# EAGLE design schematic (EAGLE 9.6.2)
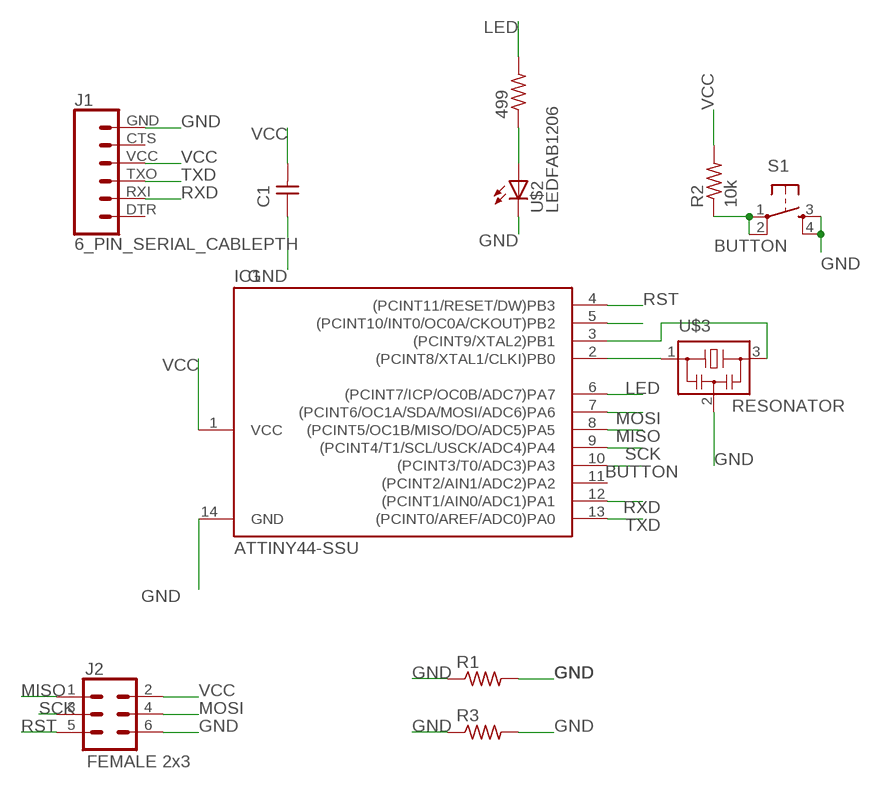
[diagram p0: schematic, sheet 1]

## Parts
499  RES-US1206FAB  [R1206FAB]
C1  CAP-UNPOLARIZEDFAB  [C1206FAB]
IC1  ATTINY44-SSU  [SOIC14]
J1  6_PIN_SERIAL_CABLEPTH  [FTDI_BASIC]
J2  FEMALE 2x3  CONN_03X2FEMALE  [2X3]
R1  RES-US1206FAB  [R1206FAB]
R2  10k  RES-US1206FAB  [R1206FAB]
R3  RES-US1206FAB  [R1206FAB]
S1  6MM_SWITCH6MM_SWITCH  [6MM_SWITCH]
U$2  LEDFAB1206  [LED1206FAB]
U$3  RESONATOR  [EFOBM]

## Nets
BUTTON: IC1.10((PCINT3/T0/ADC3)PA3) R2.1 S1.1(P) S1.2(P1)
GND: C1.1 IC1.14(GND) J1.GND J2.6 R1.1 R1.2 R3.1 R3.2 S1.3(S) S1.4(S1) U$2.2(C) U$3.2
LED: 499.2 IC1.6((PCINT7/ICP/OC0B/ADC7)PA7)
MISO: IC1.8((PCINT5/OC1B/MISO/DO/ADC5)PA5) J2.1
MOSI: IC1.7((PCINT6/OC1A/SDA/MOSI/ADC6)PA6) J2.4
N$1: IC1.5((PCINT10/INT0/OC0A/CKOUT)PB2)
N$4: IC1.2((PCINT8/XTAL1/CLKI)PB0) U$3.1
N$5: IC1.3((PCINT9/XTAL2)PB1) U$3.3
N$6: 499.1 U$2.1(A)
RST: IC1.4((PCINT11/RESET/DW)PB3) J2.5
RXD: IC1.12((PCINT1/AIN0/ADC1)PA1) J1.RXI
SCK: IC1.9((PCINT4/T1/SCL/USCK/ADC4)PA4) J2.3
TXD: IC1.13((PCINT0/AREF/ADC0)PA0) J1.TXO
VCC: C1.2 IC1.1(VCC) J1.VCC J2.2 R2.2
Unconnected: IC1.11((PCINT2/AIN1/ADC2)PA2) J1.CTS J1.DTR

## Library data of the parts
499 R1-R3 = fab:RES-US: Resistor (US Symbol)
C1 = fab:CAP-UNPOLARIZED
IC1 = fab:ATTINY44
J1 = SparkFun-Connectors:6_PIN_SERIAL_CABLE: 6-pin header connection for use with the "FTDI BASIC" pinout - CABLE SIDE. Also known as "Arduino Serial Program Header". This is used on a design to provide a 6-pin connection point for serial communication usually from a USB cable (D+/D-) to these headers (RX/TX). It also has the remaining pins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
J2 = SparkFun-Connectors:CONN_03X2: Multi connection point. Often used as Generic Header-pin footprint for 0.1 inch spaced/style header connections You can populate with any combo of single row headers, but if you'd like an exact match, check these: Header - 2x3 (Male, 0.1") (PRT-12807) Header - 2x3 (Female, 0.1") (PRT-13010) 2x3 Pin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; PROD_ID: CONN-11566
S1 = fab:6MM_SWITCH: OMRON SWITCH
U$2 = fab:LED: LED
U$3 = fab:RESONATOR

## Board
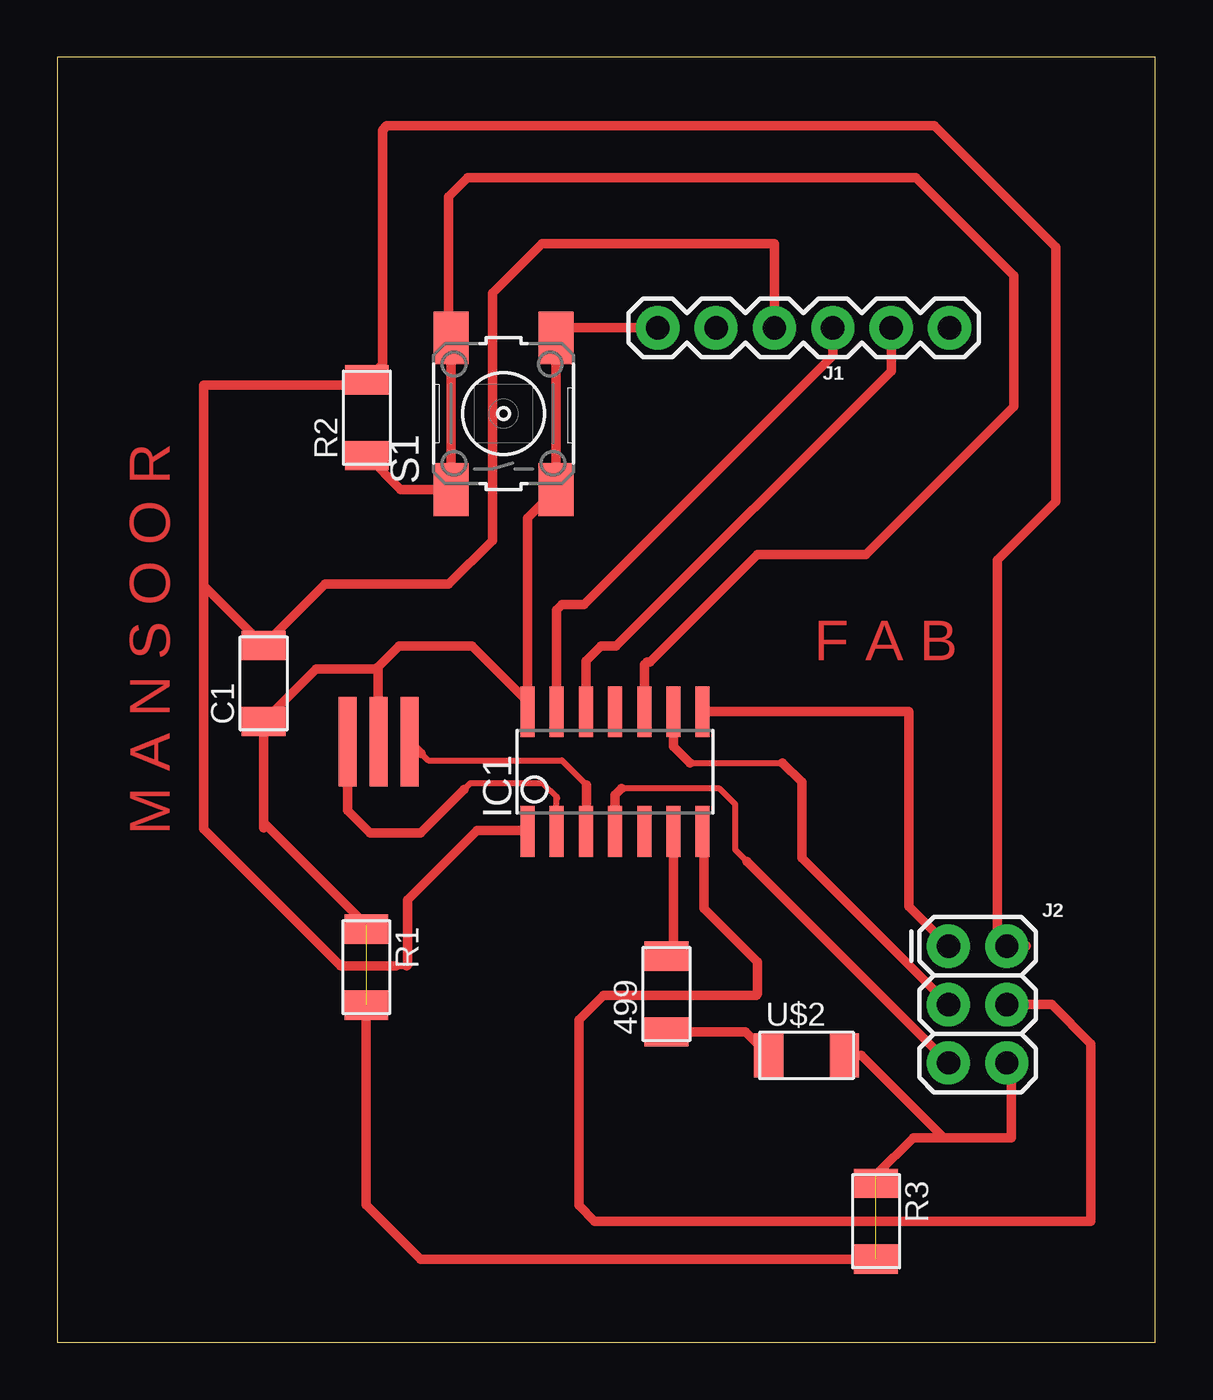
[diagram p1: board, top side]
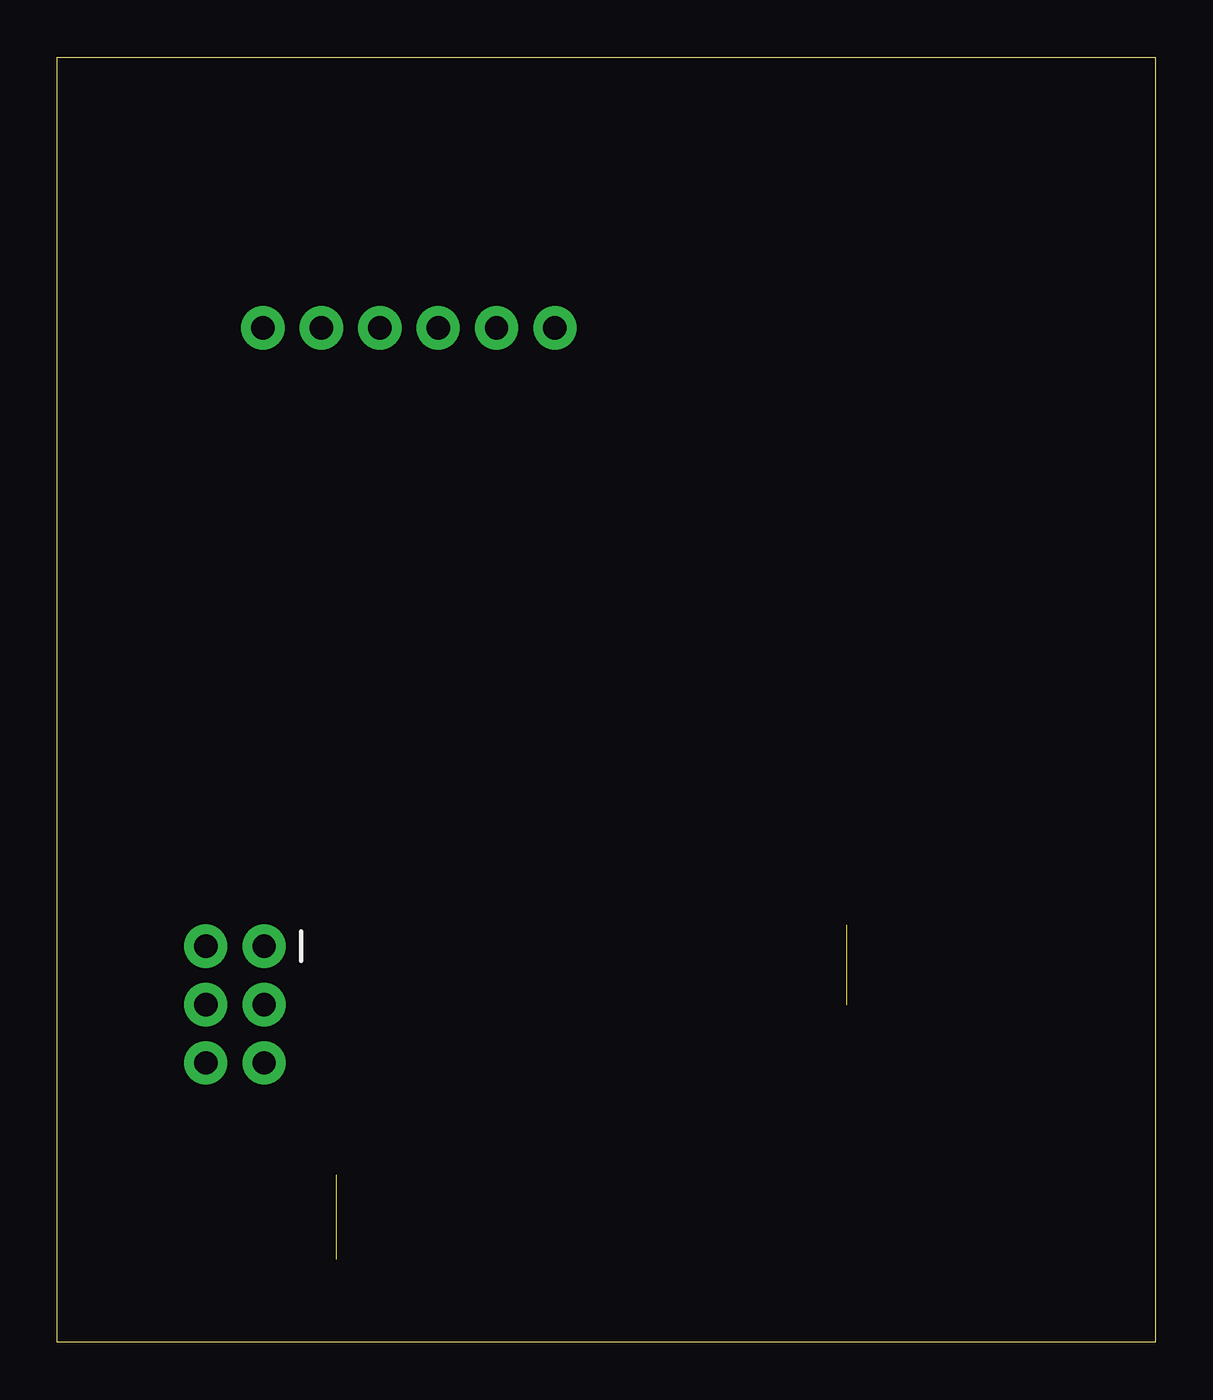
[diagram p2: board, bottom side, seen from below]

Size 47.75 x 55.88 mm. Coordinates in mm from the lower left corner, seen from the top.
Outline: 0,0 47.75,0 47.75,55.88 0,55.88 0,0
Copper layers (1*16): Top 0.035mm / dielectric 1.5mm / Bottom 0.035mm
Design rules "default *": minimum track width 6mil, minimum drill 0.35mm, track to track 16mil, track to pad 8mil, pad to pad 8mil, via to via 8mil, smd to smd 8mil, copper to edge 40mil, drill to drill 6mil, minimum pad ring 10mil, minimum via ring 8mil, stop-mask expansion 4mil, vias tented up to drill 0mil, thermal gap 10mil

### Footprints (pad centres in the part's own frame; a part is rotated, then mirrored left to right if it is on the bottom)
R1206FAB = smd 1.27 x 1.905: 1 -1.651,0; 2 1.651,0
C1206FAB = smd 1.27 x 1.905: 1 -1.651,0; 2 1.651,0
SOIC14 = smd 0.61 x 2.21: 1 -3.81,-2.603; 2 -2.54,-2.603; 3 -1.27,-2.603; 4 0,-2.603; 5 1.27,-2.603; 6 2.54,-2.603; 7 3.81,-2.603; 8 3.81,2.603; 9 2.54,2.603; 10 1.27,2.603; 11 0,2.603; 12 -1.27,2.603; 13 -2.54,2.603; 14 -3.81,2.603
FTDI_BASIC = drill 1.016 pad 1.88: CTS 10.16,0; DTR 0,0; GND 12.7,0; RXI 2.54,0; TXO 5.08,0; VCC 7.62,0
2X3 = drill 1.016 pad 1.88: 1 0,0; 2 0,2.54; 3 2.54,0; 4 2.54,2.54; 5 5.08,0; 6 5.08,2.54
6MM_SWITCH = smd 2.286 x 1.524: 1 -3.302,2.286; 2 3.302,2.286; 3 -3.302,-2.286; 4 3.302,-2.286
LED1206FAB = smd 1.27 x 1.905: 1 -1.651,0; 2 1.651,0
EFOBM = smd 0.8 x 3.9: 1 -1.35,0; 2 0,0; 3 1.35,0

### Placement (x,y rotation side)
499  26.49,15.14 90 top
C1  8.97,28.65 90 top
IC1  24.26,24.82 0 top
J1  38.81,44.12 180 top
J2  38.76,17.22 270 top
R1  13.44,16.31 270 top
R2  13.46,40.21 90 top
R3  35.61,5.26 270 top
S1  19.41,40.39 90 top
U$2  32.59,12.47 0 top
U$3  13.97,26.11 0 top

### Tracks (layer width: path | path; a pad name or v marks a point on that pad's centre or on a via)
BUTTON
  Top 0.406: 25.53,28.47 IC1.10 25.53,29.46 25.65,29.59 25.78,29.59 30.45,34.27 35.18,34.27 41.6,40.69 41.6,46.38 37.34,50.65 17.83,50.65 17,49.82 17,43.8 S1.2 | S1.2 17.12,43.92 | S1.2 S1.1 14.94,37.08 R2.1
GND  (4 unrouted)
  Top 0.406: U$3.2 13.96,26.13 13.96,29.37 | 41.81,11.63 41.5,11.94 | J1.GND 22.12,44.12 S1.4 S1.3 20.45,35.84 IC1.14 20.45,27.86 18.03,30.28 14.86,30.28 13.96,29.37 | 13.96,29.37 13.87,29.29 11.25,29.29 C1.1 8.97,22.61 | U$2.2 34.98,12.47 38.56,8.89 | 38.56,8.89 41.5,8.89 41.5,11.94 | 41.5,11.94 J2.6 | 38.56,8.89 37.24,8.89 35.61,7.26 | 8.97,22.35 8.97,22.61 | 8.97,22.61 13.44,18.14 | R1.2 13.44,5.97 15.8,3.61 R3.2
LED
  Top 0.406: 499.2 26.8,17.09 IC1.6
MISO
  Top 0.406: J2.1 37.03,18.95 37.03,27.42 IC1.8
MOSI
  Top 0.406: J2.4 43.26,14.68 44.96,12.98 44.96,5.26 23.37,5.26 22.68,5.94 22.68,14.02 23.75,15.09 30.4,15.09 30.45,15.14 30.45,16.54 28.12,18.87 28.12,22.16 IC1.7
N$4
  Top 0.254: IC1.2 21.72,23.62 | 21.72,23.62 21.74,23.65 | 21.72,23.62 21.72,23.72 21.13,24.31 17.96,24.31 17.68,24.03
  Top 0.406: U$3.1 12.63,23.13 13.61,22.15 15.8,22.15 17.68,24.03
N$5
  Top 0.254: 15.83,25.6 16.13,25.3 21.95,25.3 23.01,24.23
  Top 0.406: U$3.3 15.83,25.6 | 23.01,24.23 23.01,22.24 IC1.3
N$6
  Top 0.406: U$2.1 29.92,13.49 499.1
RST  (via drill 0.35)
  Top 0.254: 30,20.9 29.49,21.41 29.49,23.39 28.8,24.08 24.54,24.08
  Top 0.406: J2.5 30,20.9 | 24.54,24.08 24.26,23.8 IC1.4
  other vias: 38.76,12.14
RXD
  Top 0.406: 36.17,44.02 J1.RXI 36.27,42.24 24.31,30.28 23.65,30.28 22.99,29.62 IC1.12
SCK
  Top 0.254: 27.51,25.2 31.55,25.2
  Top 0.406: J2.3 32.38,21.06 32.38,24.36 31.55,25.2 | 27.51,25.2 26.8,25.91 IC1.9
TXD
  Top 0.406: J1.TXO 33.73,42.9 22.91,32.08 21.95,32.08 21.72,31.85 IC1.13
VCC
  Top 0.254: 14.73,16.36 15.19,16.36
  Top 0.406: 42.14,17.22 J2.2 40.89,17.63 40.89,34.01 43.43,36.55 43.43,47.62 38.15,52.91 14.33,52.91 14.13,52.72 14.13,42.53 R2.2 13.23,41.63 6.35,41.63 6.35,32.92 | J1.VCC 31.19,47.78 21.08,47.78 18.92,45.62 18.92,34.87 17.02,32.97 11.63,32.97 C1.2 | IC1.1 20.41,22.25 18.26,22.25 15.24,19.23 15.24,16.41 15.19,16.36 | 8.31,30.3 C1.2 | 6.35,32.92 6.35,22.33 12.32,16.36 14.73,16.36 | C1.2 6.35,32.92

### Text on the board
Top: F A B | M A N S O O R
